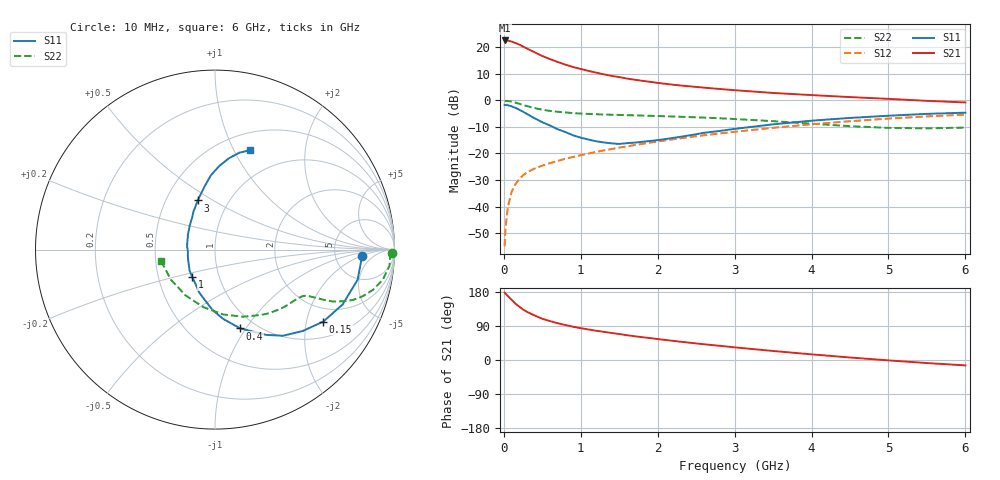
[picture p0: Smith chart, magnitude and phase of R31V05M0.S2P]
! SIEMENS Small Signal Semiconductors
! BFR181
! Si NPN RF Bipolar Junction Transistor in SOT23
! VCE = 1 V  IC = 5 mA
! Common Emitter S-Parameters:  May  1996
# GHz  S  MA  R  50
!  f  S11  S21  S12  S22
! GHz  MAG  ANG  MAG  ANG  MAG  ANG  MAG  ANG
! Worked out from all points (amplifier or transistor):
!   36 points, 10 MHz to 6 GHz, reference 50 ohm
!   highest |S21| = 22.6 dB at 10 MHz (marker M1)
!   |S21| within 3 dB of that: start of sweep to 297.2 MHz
!   unconditionally stable (mu >= 1): 907.3 MHz to 3.154 GHz
!   at 250 MHz: K = 0.45, MSG = 24.2 dB, |S12| = -28.2 dB
!   at 1.4 GHz: K = 1.09, MAG = 11.9 dB, |S12| = -18.3 dB
!   at 6 GHz: K = 0.89, MSG = 2.3 dB, |S12| = -5.4 dB
!   S11 on the Smith chart (normalised r, x): 10 MHz: 9.64, -2.20; 150 MHz: 1.49, -2.52; 400 MHz: 0.85, -0.94; 1 GHz: 0.74, -0.24; 3 GHz: 0.72, +0.43; 6 GHz: 0.69, +1.16
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0.01  0.8206 -2.6  13.43 178.0  0.0018 97.2  0.9863 -1.1
0.02  0.8166 -4.5  13.22 175.6  0.0036 87.7  0.9767 -2.1
0.05  0.8124 -11.9  13.33 169.2  0.0095 83.9  0.9766 -5.2
0.1  0.7739 -23.3  12.83 159.1  0.0188 77.7  0.9498 -10.2
0.15  0.7244 -33.6  12.01 148.9  0.0263 72.0  0.9083 -14.3
0.2  0.6666 -42.9  11.25 140.8  0.033 68.9  0.8633 -17.5
0.25  0.6114 -51.7  10.31 133.3  0.0388 65.9  0.819 -20.0
0.3  0.5552 -58.9  9.46 127.2  0.044 64.5  0.7809 -21.6
0.4  0.4608 -72.3  8.044 117.4  0.0521 61.3  0.7172 -23.8
0.5  0.3875 -83.5  6.841 108.8  0.0591 60.8  0.6667 -24.8
0.6  0.3364 -92.4  5.983 102.7  0.066 60.5  0.6333 -25.3
0.7  0.2858 -101.6  5.288 97.1  0.0723 60.8  0.6095 -25.8
0.8  0.2536 -110.6  4.705 92.3  0.0796 61.1  0.5916 -26.2
1  0.1983 -129.9  3.896 84.0  0.0929 61.9  0.5648 -27.1
1.1  0.183 -140.9  3.594 80.6  0.0997 62.4  0.5559 -27.8
1.6  0.1565 173.5  2.574 65.4  0.1363 62.4  0.5264 -32.5
2.2  0.1961 135.4  1.971 50.5  0.1849 60.8  0.4976 -40.5
3  0.2906 109.4  1.554 33.4  0.2564 55.8  0.4457 -54.7
3.5  0.354 99.7  1.379 23.8  0.3046 51.4  0.4062 -67.1
4.5  0.4672 87.0  1.153 6.6  0.4052 40.4  0.3266 -101.5
5.5  0.5574 75.8  0.98 -8.1  0.4988 27.2  0.2974 -145.7
6  0.5868 70.6  0.914 -14.2  0.5398 20.0  0.3074 -168.3
